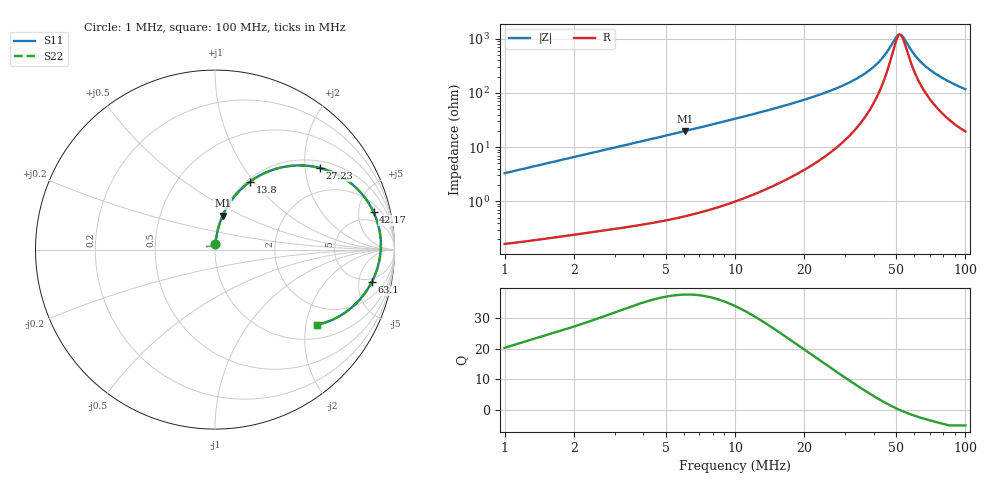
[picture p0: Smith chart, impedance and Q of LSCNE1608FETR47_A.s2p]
! LSCNE1608FETR47_A  S-PARAMETER MODEL  ( Standard Model )
! Model Generated by TAIYO YUDEN Corporation (http://www.ty-top.com)
! Version 2.0
! TAIYO YUDEN Control No. 171005
! Copyright(c) 2016 TAIYO YUDEN CO.,LTD. All Rights Reserved.
! Product Description (link to TY-COMPAS)
! https://ds.yuden.co.jp/TYCOMPAS/or/detail?pn=LSCNE1608FETR47MA&u=M
! Products Name : Inductors
! Characteristics :
!  Inductance : 0.47 [uH] , SRF(min) : - [Hz] , DC Resistance(max) : 150 [mOhm]
!  Rated Current : Saturation  2.0 [A] (dL = 30 [%]), Temp Rise  1.2 [A] (dT = 40 [degC])
!  Case Size : 1.6 x 0.8 / 0.063 x 0.031 [mm/inch] , Thickness : 0.65 / 0.026 [mm/inch]
!  (Conditions: Temperature = 25 [degC] , DC Bias Current = 0 [A])
! External Node Assignments :
!  1  o---GGG---o  2
! GND o---------o GND
! Frequency Range : 1MHz  -  100MHz  [ 402 STEP ]
# MHz S RI R 50
! Freq[MHz].  S11 Real  S11 Imag  S21 Real  S21 Imag  S12 Real  S12 Imag  S22 Real  S22 Imag
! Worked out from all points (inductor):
!   401 points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, 1 MHz to 100 MHz, reference 50 ohm
!   read as one part in series: L = 523 nH near 1.023 MHz
!   highest Q = 37.6 at 6.095 MHz (marker M1), where L = 520 nH
!   self-resonance near 52.05 MHz
!   S11 on the Smith chart (normalised r, x): 1 MHz: 1.00, +0.07; 13.8 MHz: 1.03, +0.95; 27.23 MHz: 1.19, +2.39; 42.17 MHz: 3.05, +7.28; 63.1 MHz: 4.16, -7.39; 100 MHz: 1.39, -2.31
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1  0.0027 0.0328  0.9973 -0.0328  0.9973 -0.0328  0.0027 0.0328
1.757924  0.0055 0.0571  0.9945 -0.0571  0.9945 -0.0571  0.0055 0.0571
2.818383  0.0112 0.0905  0.9888 -0.0905  0.9888 -0.0905  0.0112 0.0905
4.265795  0.0226 0.1352  0.9774 -0.1352  0.9774 -0.1352  0.0226 0.1352
6.095369  0.0429 0.1898  0.9571 -0.1898  0.9571 -0.1898  0.0429 0.1898
9.440609  0.0965 0.2813  0.9035 -0.2813  0.9035 -0.2813  0.0965 0.2813
13.80384  0.1939 0.3779  0.8061 -0.3779  0.8061 -0.3779  0.1939 0.3779
17.57924  0.2965 0.4351  0.7035 -0.4351  0.7035 -0.4351  0.2965 0.4351
22.38721  0.4395 0.468  0.5605 -0.468  0.5605 -0.468  0.4395 0.468
27.22701  0.5823 0.4555  0.4177 -0.4555  0.4177 -0.4555  0.5823 0.4555
34.27678  0.7593 0.3678  0.2407 -0.3678  0.2407 -0.3678  0.7593 0.3678
38.45918  0.8358 0.2886  0.1642 -0.2886  0.1642 -0.2886  0.8358 0.2886
42.16965  0.8832 0.2098  0.1168 -0.2098  0.1168 -0.2098  0.8832 0.2098
50.69907  0.9242 0.0268  0.0758 -0.0268  0.0758 -0.0268  0.9242 0.0268
51.88  0.9237 0.00331  0.0763 -0.00331  0.0763 -0.00331  0.9237 0.00331
53.08844  0.9219 -0.0201  0.0781 0.0201  0.0781 0.0201  0.9219 -0.0201
58.88437  0.8994 -0.1209  0.1006 0.1209  0.1006 0.1209  0.8994 -0.1209
63.09573  0.8729 -0.182  0.1271 0.182  0.1271 0.182  0.8729 -0.182
67.6083  0.8392 -0.2371  0.1608 0.2371  0.1608 0.2371  0.8392 -0.2371
74.98942  0.7781 -0.3075  0.2219 0.3075  0.2219 0.3075  0.7781 -0.3075
84.13951  0.699 -0.3676  0.301 0.3676  0.301 0.3676  0.699 -0.3676
100  0.5682 -0.418  0.4318 0.418  0.4318 0.418  0.5682 -0.418
